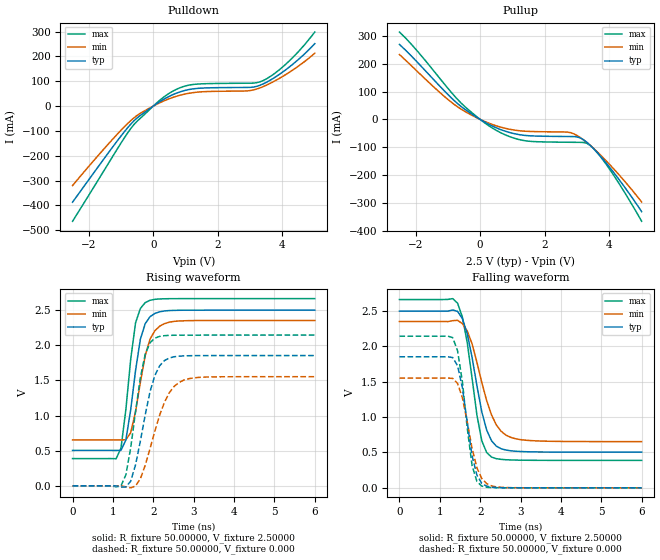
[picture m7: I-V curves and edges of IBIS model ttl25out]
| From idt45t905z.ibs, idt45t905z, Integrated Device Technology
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|   Model ttl25out
[Model]   ttl25out
Model_type   Output
Polarity   Non-Inverting
Vmeas =  1.25000V
C_comp   5.00000pF   5.00000pF   5.00000pF
[Temperature Range]   45.00000   0.14000k   -30.00000
[Voltage Range]   2.50000V   2.30000V   2.70000V
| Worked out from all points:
|   slope of the pulldown table from 0 to 0.375 V, typ, clamps not added: 12.1 ohm
|   slope of the pullup table from 0 to 0.375 V, typ, clamps not added: 15.8 ohm
|   rising waveform, R_fixture 50.00000, V_fixture 2.50000: 20-80 % time 297ps typ, 346ps min, 268ps max; typ from 0.505 V to 2.5 V
|   rising waveform, R_fixture 50.00000, V_fixture 0.000: 20-80 % time 408ps typ, 515ps min, 338ps max; typ from 0 V to 1.85 V
|   falling waveform, R_fixture 50.00000, V_fixture 2.50000: 20-80 % time 412ps typ, 503ps min, 353ps max; typ from 2.5 V to 0.505 V
|   falling waveform, R_fixture 50.00000, V_fixture 0.000: 20-80 % time 301ps typ, 337ps min, 273ps max; typ from 1.85 V to 0 V
[Pulldown]
| voltage   I(typ)   I(min)   I(max)
-2.5V     -387.1mA   -320.1mA   -464mA
-1.3V     -172.3mA   -139.4mA   -211.9mA
-700mV    -73.11mA   -58.92mA   -90.86mA
-400mV    -37.65mA   -28.88mA   -48.96mA
300mV     25.63mA    19.24mA    33.79mA
700mV     51.07mA    38.83mA    66.42mA
1.1V      66.37mA    51.46mA    84.22mA
2.9V      74.99mA    61.06mA    92.02mA
3.4V      89.1mA     78.19mA    102.5mA
4.1V      145.9mA    126.7mA    168.2mA
4.5V      188.2mA    161.4mA    220mA
5V        251.4mA    212.9mA    298.1mA
[Pullup]
| voltage   I(typ)   I(min)   I(max)
-2.5V     269.9mA    233.5mA    314.3mA
-800mV    67.39mA    53.61mA    84.83mA
-300mV    22.62mA    17.64mA    28.64mA
400mV     -25.11mA   -19.06mA   -32.59mA
900mV     -46.72mA   -35.05mA   -61.28mA
1.4V      -57.66mA   -42.47mA   -76.9mA
2.8V      -61.54mA   -47.61mA   -82.16mA
3.1V      -66.62mA   -65.23mA   -82.46mA
3.4V      -92.17mA   -92.61mA   -92.89mA
3.7V      -128.7mA   -125.1mA   -129.7mA
4.1V      -185.6mA   -173.4mA   -194.7mA
5V        -331.7mA   -297.2mA   -366.3mA
[Ramp]
| variable   typ   min   max
dV/dt_r   1.11240/0.40540n   0.93180/0.51638n   1.28700/0.32701n
dV/dt_f   1.19718/0.40789n   1.02540/0.47741n   1.36518/0.35300n
R_load = 50.00000
[Rising Waveform]
R_fixture = 50.00000
V_fixture = 2.50000
C_fixture = 0.000F
R_dut = 2.40000m
L_dut = 0.90000nH
C_dut = 60.00000fF
| time   V(typ)   V(min)   V(max)
0s        504.8mV    653.9mV    388.4mV
1.08ns    504.7mV    653.9mV    386.6mV
1.2ns     506.3mV    653.7mV    539.2mV
1.32ns    652.2mV    656.5mV    1.083V
1.44ns    1.082V     757.3mV    1.799V
1.56ns    1.639V     1.056V     2.318V
1.8ns     2.308V     1.853V     2.607V
2.04ns    2.454V     2.208V     2.654V
2.4ns     2.494V     2.329V     2.663V
6ns       2.5V       2.353V     2.664V
[Rising Waveform]
R_fixture = 50.00000
V_fixture = 0.000
C_fixture = 0.000F
R_dut = 2.40000m
L_dut = 0.90000nH
C_dut = 60.00000fF
| time   V(typ)   V(min)   V(max)
0s        0V         0V         0V
1.2ns     -15.93mV   -14.73uV   745uV
1.32ns    -16.19mV   -13.53mV   156.8mV
1.44ns    66.38mV    -27.62mV   540.4mV
1.68ns    639mV      101.2mV    1.542V
1.8ns     1.011V     293.9mV    1.873V
2.04ns    1.573V     781.8mV    2.102V
2.4ns     1.819V     1.329V     2.142V
2.76ns    1.849V     1.506V     2.144V
6ns       1.854V     1.553V     2.145V
[Falling Waveform]
R_fixture = 50.00000
V_fixture = 2.50000
C_fixture = 0.000F
R_dut = 2.40000m
L_dut = 0.90000nH
C_dut = 60.00000fF
| time   V(typ)   V(min)   V(max)
0s        2.5V       2.353V     2.664V
1.44ns    2.497V     2.37V      2.612V
1.56ns    2.393V     2.322V     2.416V
1.68ns    2.18V      2.219V     2.054V
1.92ns    1.444V     1.774V     1.028V
2.04ns    1.075V     1.492V     666.2mV
2.28ns    667.3mV    1.033V     435.9mV
2.52ns    552.7mV    799.5mV    402.6mV
2.88ns    517.9mV    694.1mV    392.5mV
6ns       504.8mV    653.9mV    388.4mV
[Falling Waveform]
R_fixture = 50.00000
V_fixture = 0.000
C_fixture = 0.000F
R_dut = 2.40000m
L_dut = 0.90000nH
C_dut = 60.00000fF
| time   V(typ)   V(min)   V(max)
0s        1.854V     1.553V     2.145V
1.32ns    1.843V     1.548V     2.125V
1.44ns    1.728V     1.476V     1.939V
1.56ns    1.416V     1.274V     1.5V
1.68ns    923.4mV    932.4mV    843mV
1.8ns     451.6mV    556.4mV    314.5mV
1.92ns    177.3mV    281.9mV    89.2mV
2.04ns    63.41mV    130.8mV    24.09mV
2.52ns    2.361mV    6.883mV    945.9uV
6ns       679.4nV    2.744uV    0V
